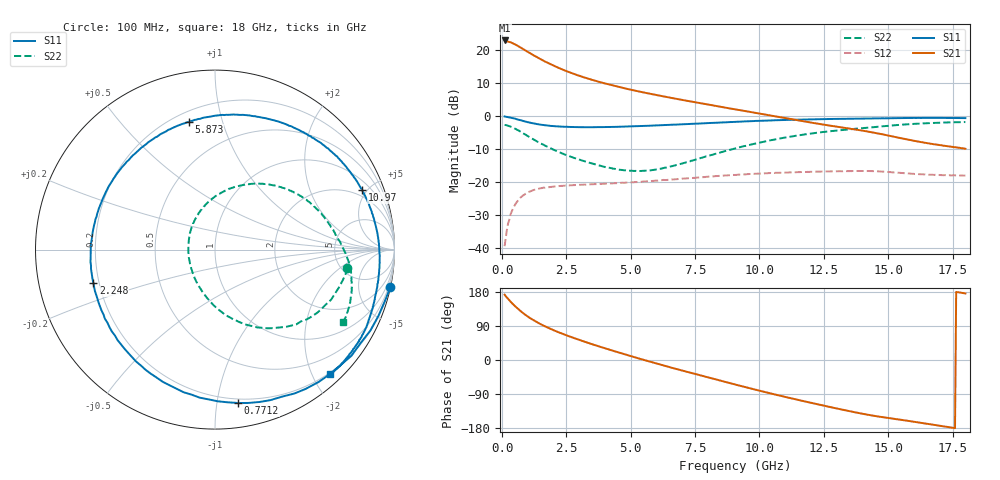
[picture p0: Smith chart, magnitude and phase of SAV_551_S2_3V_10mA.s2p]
! Data provided by Modelithics, Inc.  Tampa, Florida USA, June 2008
!Model SAV-551+
!VAR V_out= 3
!VAR I_out= 10
!VAR V_in= 0.2923
!VAR I_in= 0.8631
!BEGIN ACDATA
# GHZ S MA R 50
! Scattering Parameters
!% F n11x n11y n21x n21y n12x n12y n22x n22y
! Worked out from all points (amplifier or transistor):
!   401 points, 100 MHz to 18 GHz, reference 50 ohm
!   highest |S21| = 23.0 dB at 100 MHz (marker M1)
!   |S21| within 3 dB of that: start of sweep to 903 MHz
!   unconditionally stable (mu >= 1): 4.821 GHz to 10.32 GHz
!   at 3.054 GHz: K = 0.71, MSG = 16.5 dB, |S12| = -20.7 dB
!   at 9.05 GHz: K = 1.08, MAG = 8.2 dB, |S12| = -17.8 dB
!   at 18 GHz: K = 0.85, MSG = 4.1 dB, |S12| = -17.9 dB
!   lowest NFmin = 0.08 dB at 500 MHz
!   S11 on the Smith chart (normalised r, x): 100 MHz: 0.04, -9.38; 771.2 MHz: 0.17, -1.15; 2.248 GHz: 0.18, -0.13; 5.873 GHz: 0.26, +0.78; 10.97 GHz: 1.51, +4.65; 18 GHz: 0.18, -2.28
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0.1  0.999 -12.2  14.19 172.4  0.0108 82.7  0.7423 -7.8
0.1895  0.9823 -22.3  13.74 164.8  0.01917 77.3  0.7319 -13.5
0.279  0.9643 -32.5  13.44 157.6  0.02677 68.2  0.7128 -20.0
0.3685  0.9501 -42.9  13.11 151.1  0.03568 64.8  0.6895 -26.3
0.458  0.9368 -51.9  12.6 145.3  0.04257 60.8  0.669 -31.8
0.59225  0.9002 -65.5  11.83 136.5  0.05127 53.9  0.6242 -39.8
0.77125  0.8644 -81.4  10.79 126.2  0.06124 46.2  0.5711 -49.2
0.9055  0.836 -92.2  10.03 119.2  0.06717 40.6  0.5326 -55.4
1.0845  0.8042 -105.5  9.102 110.7  0.07288 34.7  0.4825 -63.0
1.39775  0.7631 -125.1  7.746 98.3  0.07974 26.3  0.4093 -73.8
1.8005  0.7244 -145.8  6.413 84.6  0.08447 18.1  0.3412 -85.5
2.248  0.7027 -164.5  5.34 71.8  0.08829 11.3  0.2841 -96.7
3.09825  0.6862 167.0  4.012 50.8  0.092 2.0  0.2153 -116.4
4.396  0.694 133.1  2.886 22.6  0.09726 -8.3  0.16 -150.6
5.87275  0.7261 101.6  2.159 -6.8  0.1054 -18.0  0.1544 161.3
6.0965  0.7338 97.4  2.076 -11.0  0.1072 -19.6  0.1599 154.1
7.439  0.774 73.9  1.655 -36.0  0.1173 -29.6  0.2167 116.0
9.05  0.8258 49.0  1.281 -64.5  0.1295 -43.4  0.3268 81.7
10.97425  0.8849 22.1  0.9445 -96.9  0.1409 -63.6  0.4762 49.2
12.04825  0.9045 8.7  0.8014 -113.7  0.1445 -75.3  0.5532 33.9
15.0465  0.9388 -22.6  0.509 -153.5  0.1434 -105.9  0.7238 -1.1
18  0.9438 -47.2  0.3236 175.6  0.1271 -131.4  0.8209 -29.3
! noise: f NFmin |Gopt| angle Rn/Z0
0.5  0.084  0.3777  24.24  0.093
0.7  0.119  0.3927  34.11  0.084
0.9  0.154  0.4072  43.86  0.077
1  0.171  0.4142  48.68  0.073
1.9  0.328  0.471  90.69  0.05
2.4  0.415  0.4975  112.9  0.044
3  0.519  0.5248  138.5  0.043
3.9  0.675  0.5561  174.8  0.056
5  0.867  0.5789  -144.3  0.093
6  1.041  0.5847  -110.5  0.147
